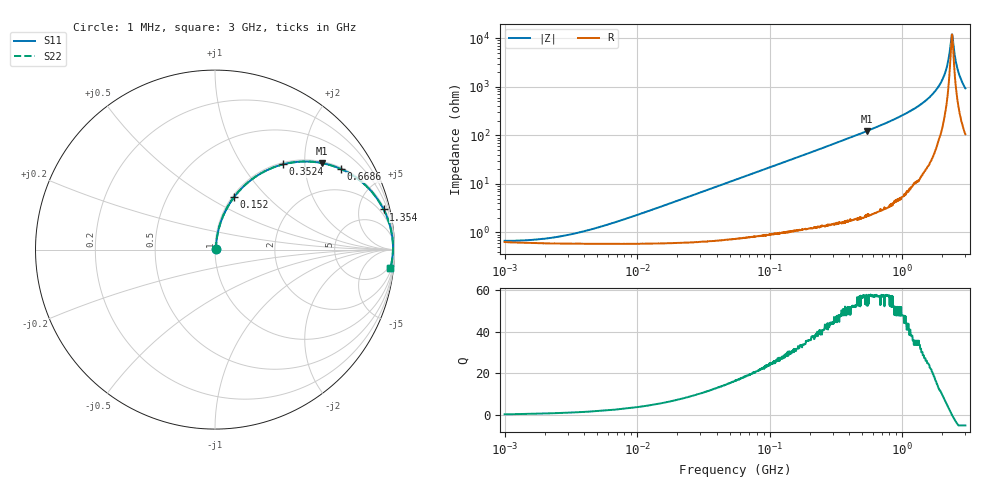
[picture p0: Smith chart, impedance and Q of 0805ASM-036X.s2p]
!s-Parameter Generated by FASTRON Sdn. Bhd.
!FASTRON P/N : 0805ASM-036X
!Keysight Technologies: E4991B_MY54100416_A.01.15
!Date: Fri Jun 19 14:48:48 2026
!Version  :Rev00  Fri Jun 19 14:48:48 2026
!Data & Calibration Information:
!Freq  S11  S21  S12  S22
!PortZ  Port1:50+j0  Port2:50+j0
!When reading reference impedance value at option line is always used.
! Remarks : This data is being provided solely for informational purposes.
# Hz S dB R 50
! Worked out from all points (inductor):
!   1601 points, 1 MHz to 3 GHz, reference 50 ohm
!   read as one part in series: L = 35.4 nH near 7.898 MHz
!   highest Q = 57.4 at 539.2 MHz (marker M1), where L = 35.9 nH
!   self-resonance near 2.371 GHz
!   S11 on the Smith chart (normalised r, x): 1 MHz: 1.01, +0.00; 152 MHz: 1.02, +0.66; 352.4 MHz: 1.03, +1.55; 668.6 MHz: 1.06, +3.10; 1.354 GHz: 1.24, +8.33; 3 GHz: 3, -18
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1000000  -43.50 19.0  -0.06 -0.1  -0.06 -0.1  -43.50 19.0
1955280  -42.70 35.7  -0.05 -0.2  -0.05 -0.2  -42.70 35.7
3804036  -39.80 54.8  -0.05 -0.5  -0.05 -0.5  -39.80 54.8
1.447069e7  -29.80 77.7  -0.06 -1.8  -0.06 -1.8  -29.80 77.7
5.504702e7  -18.40 79.7  -0.13 -6.9  -0.13 -6.9  -18.40 79.7
1.520175e8  -10.10 70.0  -0.54 -18.2  -0.54 -18.2  -10.10 70.0
2.083556e8  -7.75 64.3  -0.90 -24.2  -0.90 -24.2  -7.75 64.3
3.523638e8  -4.34 51.5  -2.13 -37.3  -2.13 -37.3  -4.34 51.5
5.391547e8  -2.31 39.0  -4.02 -50.0  -4.02 -50.0  -2.31 39.0
6.685918e8  -1.58 32.5  -5.39 -56.5  -5.39 -56.5  -1.58 32.5
7.925923e8  -1.13 27.6  -6.70 -61.4  -6.70 -61.4  -1.13 27.6
1.353887e9  -0.30 13.4  -12.70 -74.9  -12.70 -74.9  -0.30 13.4
1.67892e9  -0.15 8.2  -16.90 -79.0  -16.90 -79.0  -0.15 8.2
1.970482e9  -0.09 4.5  -22.00 -80.2  -22.00 -80.2  -0.09 4.5
2.156205e9  -0.07 2.4  -27.50 -77.4  -27.50 -77.4  -0.07 2.4
2.312676e9  -0.07 0.7  -36.80 -55.9  -36.80 -55.9  -0.07 0.7
2.371269e9  -0.07 0.1  -41.60 -9.5  -41.60 -9.5  -0.07 0.1
2.443543e9  -0.07 -0.7  -36.90 52.9  -36.90 52.9  -0.07 -0.7
2.556106e9  -0.08 -1.8  -29.80 71.9  -29.80 71.9  -0.08 -1.8
2.673854e9  -0.10 -2.9  -25.70 76.3  -25.70 76.3  -0.10 -2.9
2.853575e9  -0.12 -4.7  -21.70 77.7  -21.70 77.7  -0.12 -4.7
3e9  -0.15 -6.1  -19.50 77.4  -19.50 77.4  -0.15 -6.1
